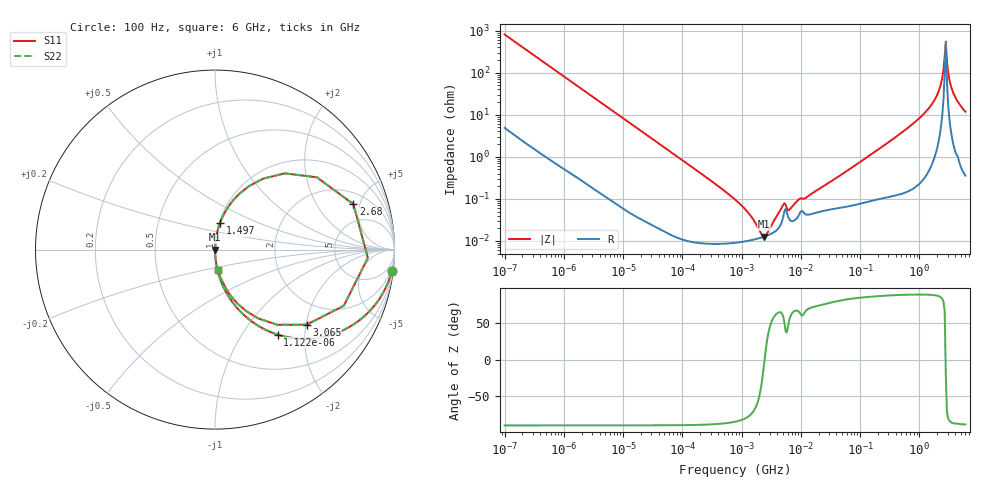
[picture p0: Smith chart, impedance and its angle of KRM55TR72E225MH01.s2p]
!Murata Part Number: KRM55TR72E225MH01
!These Parameters are Measured in Series Mode Connection
!Data Generated on Jan 08, 2026
!  o--ll--o
!Port1  Port2
!  o------o
!Operation Temp=25[degC], DC Bias Voltage=0[V]
!Freq. Start=100[Hz] Stop=6[GHz] 401[Steps]
# Hz S RI R 50
!Freq.(Hz) S11(Real) S11(Imag) S21(Real) S21(Imag) S12(Real) S12(Imag) S22(Real) S22(Imag)
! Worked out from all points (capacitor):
!   401 points, 100 Hz to 6 GHz, reference 50 ohm
!   read as one part in series: C = 1.96 uF near 109 Hz
!   lowest |Z| = 12.7 mohm at 2.373 MHz (marker M1)
!   series resonance near 2.446 MHz, so ESL is about 2.2 nH
!   S11 on the Smith chart (normalised r, x): 100 Hz: 1, -16; 1.122 kHz: 1.01, -1.46; 1.497 GHz: 1.01, +0.30; 2.68 GHz: 2.93, +4.34; 3.065 GHz: 1.36, -2.02; 6 GHz: 1.01, -0.24
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100  0.9843 -0.1212  0.0157 0.1212  0.0157 0.1212  0.9843 -0.1212
350  0.8427 -0.3611  0.1573 0.3611  0.1573 0.3611  0.8427 -0.3611
1122  0.3484 -0.4733  0.6516 0.4733  0.6516 0.4733  0.3484 -0.4733
2008  0.1448 -0.3486  0.8552 0.3486  0.8552 0.3486  0.1448 -0.3486
7358  0.0132 -0.1106  0.9868 0.1106  0.9868 0.1106  0.0132 -0.1106
40335  0.000618 -0.0206  0.9994 0.0206  0.9994 0.0206  0.000618 -0.0206
774597  9.08e-05 -0.000962  0.9999 0.000962  0.9999 0.000962  9.08e-05 -0.000962
1325623  0.000102 -0.000438  0.9999 0.000438  0.9999 0.000438  0.000102 -0.000438
2372521  0.000125 -2.03e-05  0.9999 2.03e-05  0.9999 2.03e-05  0.000125 -2.03e-05
5079039  0.000393 0.000617  0.9996 -0.000617  0.9996 -0.000617  0.000393 0.000617
6644369  0.000305 0.000493  0.9997 -0.000493  0.9997 -0.000493  0.000305 0.000493
9090158  0.00039 0.000865  0.9996 -0.000865  0.9996 -0.000865  0.00039 0.000865
1.555665e7  0.000441 0.00128  0.9996 -0.00128  0.9996 -0.00128  0.000441 0.00128
3.124326e8  0.00164 0.0229  0.9984 -0.0229  0.9984 -0.0229  0.00164 0.0229
1.497423e9  0.0271 0.1466  0.9729 -0.1466  0.9729 -0.1466  0.0271 0.1466
2.142435e9  0.1402 0.3151  0.8598 -0.3151  0.8598 -0.3151  0.1402 0.3151
2.450438e9  0.3885 0.4247  0.6115 -0.4247  0.6115 -0.4247  0.3885 0.4247
2.679998e9  0.7709 0.2531  0.2291 -0.2531  0.2291 -0.2531  0.7709 0.2531
3.065283e9  0.5111 -0.4182  0.4889 0.4182  0.4889 0.4182  0.5111 -0.4182
3.352442e9  0.2422 -0.384  0.7578 0.384  0.7578 0.384  0.2422 -0.384
3.8344e9  0.0988 -0.2713  0.9012 0.2713  0.9012 0.2713  0.0988 -0.2713
6e9  0.0173 -0.1162  0.9827 0.1162  0.9827 0.1162  0.0173 -0.1162
